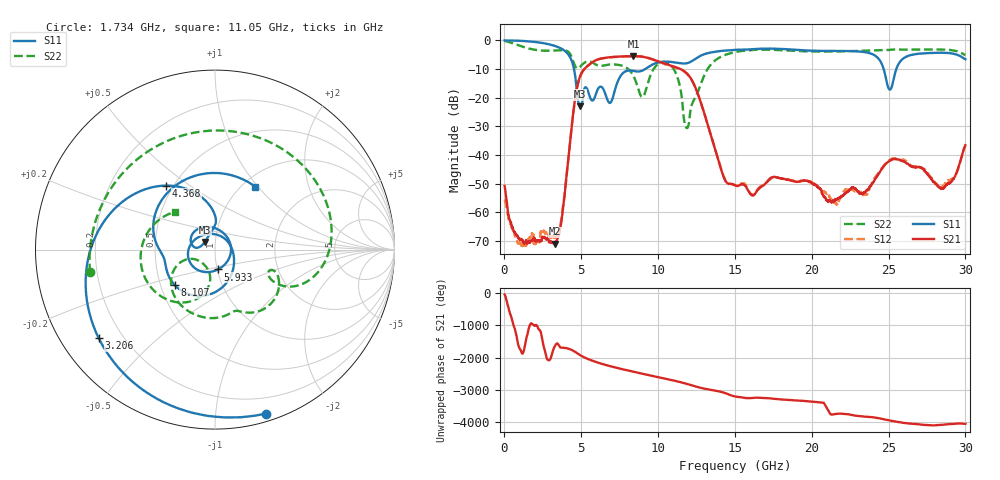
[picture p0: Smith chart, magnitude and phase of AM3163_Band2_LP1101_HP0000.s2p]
!Agilent Technologies,E8364B,MY43040894,A.07.50.67
!Agilent E8364B: A.07.50.67
!Date: Thursday, August 20, 2020 12:03:15
!Correction: S11(Full 2 Port(1,2))
!S21(Full 2 Port(1,2))
!S12(Full 2 Port(1,2))
!S22(Full 2 Port(1,2))
!S2P File: Measurements: S11, S21, S12, S22:
# Hz S  dB  R 50
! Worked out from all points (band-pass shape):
!   3201 points, 10 MHz to 30 GHz, reference 50 ohm
!   highest |S21| = -5.49 dB at 8.398 GHz (marker M1); lowest = -70.9 dB at 3.281 GHz (marker M2)
!   |S21| within 3 dB of the highest: 5.502 GHz to 10.65 GHz (5.147 GHz wide, 63.7 % of centre)
!   lowest |S11| = -22.9 dB at 4.94 GHz (marker M3), VSWR 1.15, Z = 44.4 + j3.79 ohm
!   |S11| at or under -10 dB: 4.528 GHz to 9.155 GHz (4.627 GHz wide, 67.6 % of centre); 24.68 GHz to 25.5 GHz (818.6 MHz wide, 3.26 % of centre)
!   |S22| runs from -30.6 to -0.2 dB; largest |S21 - S12| = 0.0077
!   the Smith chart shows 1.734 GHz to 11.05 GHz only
!   S11 on the Smith chart (normalised r, x): 1.734 GHz: 0.06, -1.36; 3.206 GHz: 0.11, -0.33; 4.368 GHz: 0.46, +0.41; 5.933 GHz: 1.01, -0.23; 8.107 GHz: 0.59, -0.26; 11.05 GHz: 1.14, +0.97
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1e7  -0.00 -2.8  -50.73 -54.1  -55.46 52.5  -0.21 -7.9
7.878656e8  -0.08 -32.5  -67.89 104.4  -69.59 -19.2  -1.45 -84.7
1.734425e9  -0.39 -72.7  -69.97 140.5  -68.20 -43.2  -3.00 -169.6
3.205809e9  -1.78 -142.6  -70.89 80.8  -68.63 -34.2  -3.52 77.4
3.280784e9  -1.91 -146.8  -70.95 154.4  -68.93 -5.6  -3.49 71.8
4.367922e9  -6.98 127.2  -30.42 38.7  -30.41 38.1  -5.70 -21.9
4.939606e9  -22.93 143.5  -12.30 -127.2  -12.30 -127.5  -9.10 -19.7
5.014581e9  -22.54 158.3  -11.43 -147.9  -11.44 -148.2  -8.64 -21.4
5.933025e9  -19.02 -81.7  -6.96 29.2  -6.98 29.0  -8.37 -65.7
6.832725e9  -21.79 65.1  -5.88 -98.5  -5.92 -98.6  -8.39 -88.9
8.1073e9  -10.48 -138.9  -5.51 115.6  -5.51 115.8  -10.25 -142.9
8.397828e9  -10.64 -155.8  -5.49 84.5  -5.47 84.6  -12.44 -156.1
1.000979e10  -7.67 129.3  -7.30 -84.9  -7.40 -85.5  -8.18 -135.6
1.105007e10  -7.62 57.2  -9.17 168.9  -9.31 169.4  -10.29 136.6
1.187479e10  -7.94 12.8  -11.51 68.2  -11.63 69.1  -30.59 138.9
1.5005e10  -3.28 -136.9  -50.56 41.4  -50.46 41.5  -4.08 -168.6
1.781656e10  -2.90 97.5  -47.94 -44.3  -47.92 -44.9  -3.35 66.4
2.000958e10  -3.57 -13.4  -49.78 -119.3  -49.62 -122.4  -3.85 -25.4
2.354278e10  -4.15 -148.6  -52.40 135.1  -53.46 134.9  -3.55 -135.0
2.500479e10  -16.75 176.1  -42.23 28.5  -41.98 29.8  -3.33 -172.0
2.850987e10  -4.28 105.2  -51.57 -110.1  -50.87 -111.0  -3.19 95.6
3e10  -6.56 48.0  -36.53 -84.1  -36.80 -83.9  -5.07 51.6
